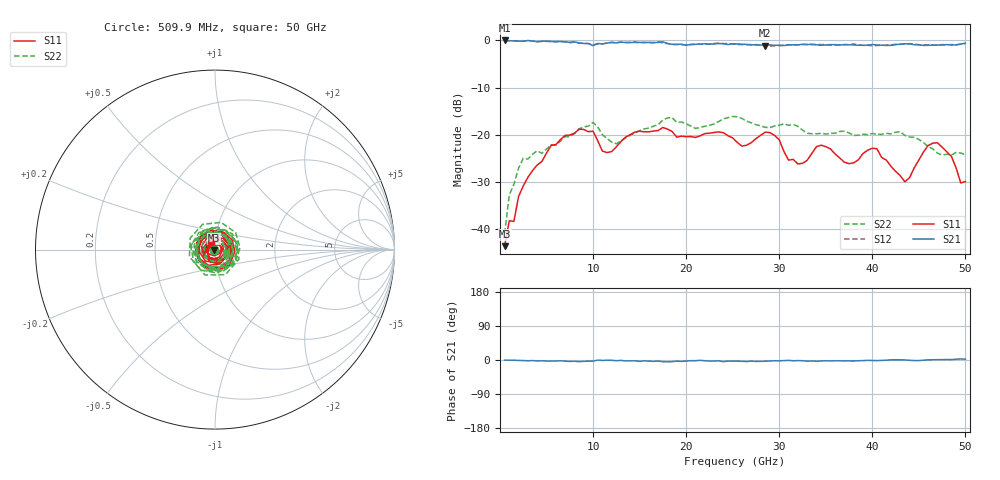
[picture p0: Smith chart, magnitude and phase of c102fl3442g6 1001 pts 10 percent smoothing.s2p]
! 8/14/2019 7:26:52 AM
! Y:\TERRY-ANALYZER-FILES\CONICAL DATA FOR CLAUDE\C102FL3442G6 1001 PTS 10 PERCENT SMOOTHING.S2P
! CHANNEL.1
! TR.MEASUREMENT
! CORRECTED.DATA
# GHZ S RI R 50.0
! FREQ.GHZ  S11RE  S11IM  S21RE  S21IM  S12RE  S12IM  S22RE  S22IM
!; PortSelection: Port_12
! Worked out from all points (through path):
!   100 points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, 509.9 MHz to 50 GHz, reference 50 ohm
!   highest |S21| = 0.00 dB at 509.9 MHz (marker M1); lowest = -1.1 dB at 28.5 GHz (marker M2)
!   lowest |S11| = -43.6 dB at 509.9 MHz (marker M3), VSWR 1.01, Z = 49.4 - j0.328 ohm
!   |S11| at or under -10 dB: start of sweep to end of sweep
!   |S22| runs from -40.9 to -16.1 dB; largest |S21 - S12| = 0.033
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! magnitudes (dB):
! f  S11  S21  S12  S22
! 509.9 MHz  -43.6  0.0  0.0  -40.9
! 1.01 GHz  -38.2  -0.1  -0.1  -32.7
! 1.51 GHz  -38.3  -0.1  -0.1  -30.5
! 2.51 GHz  -30.8  -0.2  -0.2  -25.0
! 5.509 GHz  -22.2  -0.2  -0.2  -22.1
! 9.008 GHz  -18.9  -0.6  -0.6  -18.3
! 10.01 GHz  -19.2  -1.1  -0.9  -17.4
! 11.51 GHz  -23.7  -0.6  -0.6  -20.8
! 17.51 GHz  -18.4  -0.3  -0.6  -16.8
! 21.01 GHz  -20.5  -0.8  -0.8  -18.6
! 25.5 GHz  -21.6  -0.8  -0.9  -16.2
! 28.5 GHz  -19.4  -1.1  -1.0  -18.4
! 30 GHz  -21.0  -1.0  -1.1  -18.0
! 31 GHz  -25.4  -1.0  -0.9  -18.0
! 33.5 GHz  -23.9  -0.8  -0.9  -19.8
! 34.5 GHz  -22.2  -1.0  -0.9  -19.7
! 37.5 GHz  -26.1  -0.9  -0.9  -19.6
! 40.5 GHz  -22.9  -1.0  -1.1  -19.8
! 42 GHz  -26.6  -1.0  -0.9  -19.8
! 43.5 GHz  -29.9  -0.7  -0.8  -20.1
! 47 GHz  -21.7  -1.0  -1.0  -23.9
! 50 GHz  -29.9  -0.6  -0.7  -24.2
